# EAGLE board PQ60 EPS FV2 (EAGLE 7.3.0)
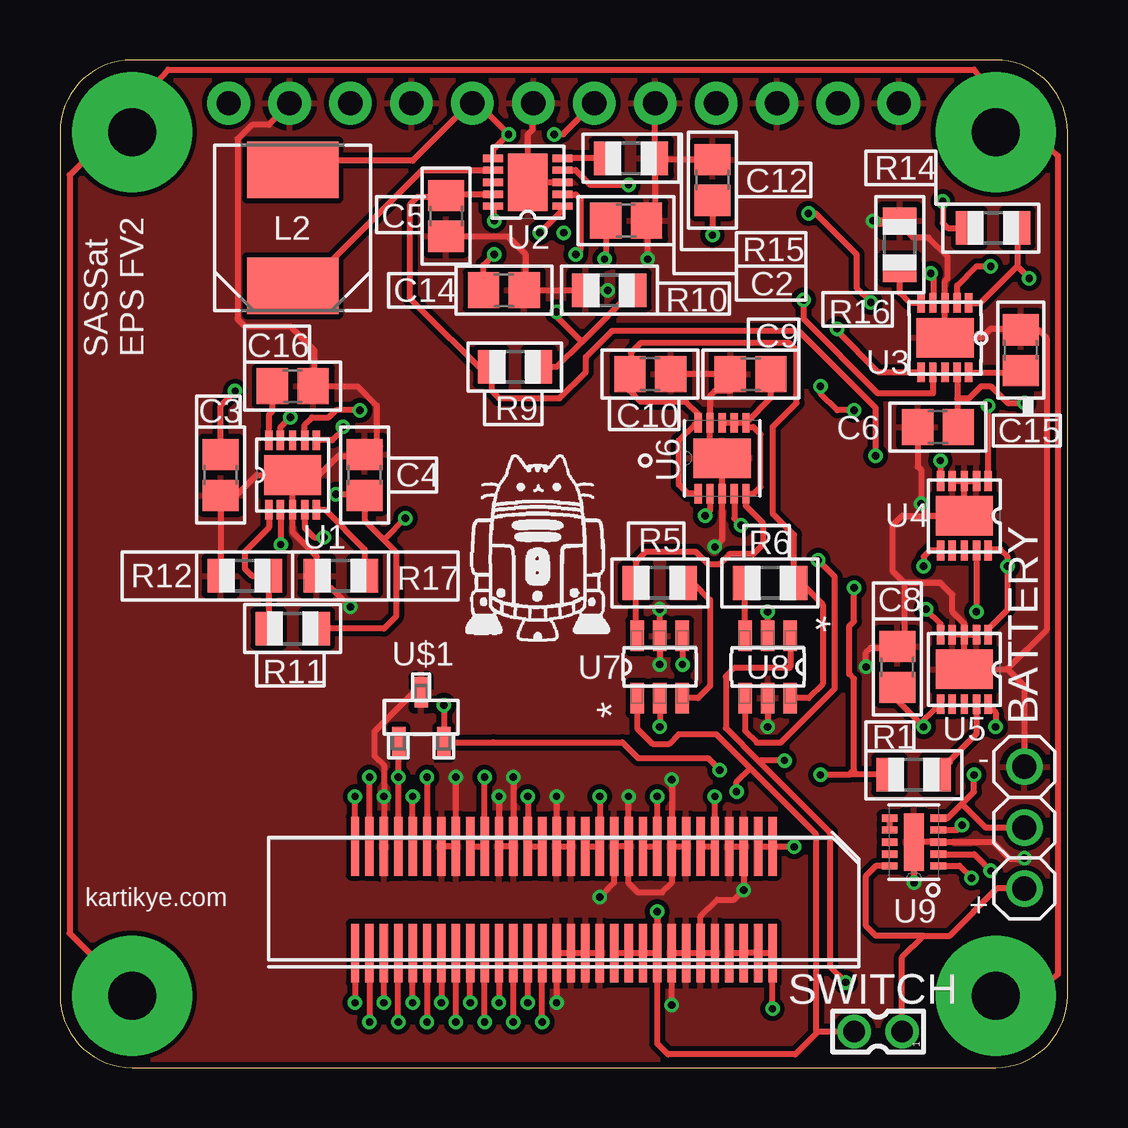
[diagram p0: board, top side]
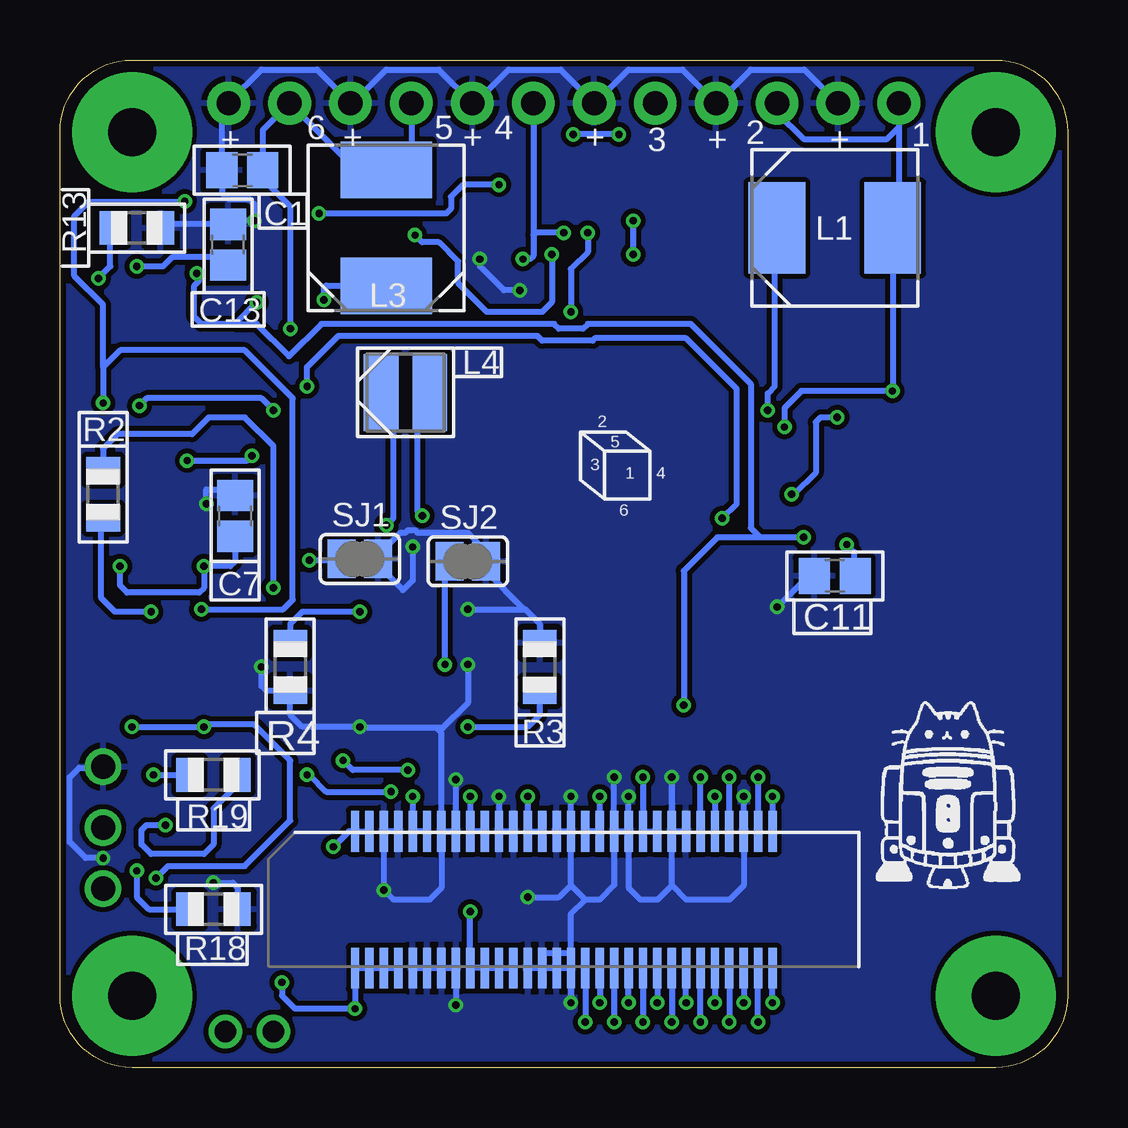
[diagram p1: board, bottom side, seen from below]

Size 42 x 42 mm. Coordinates in mm from the lower left corner, seen from the top.
Outline: 42,3 42,39 arc90 39,42 3,42 arc90 0,39 0,3 arc90 3,0 39,0 arc90 42,3
Copper layers (1*16): Top 0.035mm / dielectric 1.5mm / Bottom 0.035mm
Design rules "SeeedStudio_2layer_DRU_no_angle_20140221 *": minimum track width 6mil, minimum drill 0.3mm, track to track 6mil, track to pad 6mil, pad to pad 6mil, via to via 6mil, smd to smd 0mil, copper to edge 10mil, drill to drill 10mil, minimum pad ring 10mil, minimum via ring 6mil, stop-mask expansion 2mil, vias tented up to drill 100mil, thermal gap 10mil
Net classes: 0 default: clearance 0.205 mm

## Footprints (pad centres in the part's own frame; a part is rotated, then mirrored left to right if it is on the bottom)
1X03 = drill 1.016: 1 -2.54,0; 2 0,0; 3 2.54,0
C0805 = smd 1.3 x 1.5: 1 -0.85,0; 2 0.85,0
IND_ELL6XH = smd 2.362 x 3.81: 1 -2.413,0; 2 2.413,0
IND_ELL3FU = smd 1.448 x 3.2: 1 -1.016,0; 2 1.016,0
R0805 = smd 1.1 x 1.4: 1 -1,0; 2 1,0
SJ = smd 1.168 x 1.6: 1 -0.762,0; 2 0.762,0
1X12-CB = drill 1.016 pad 1.778: 1 -13.97,0; 2 -11.43,0; 3 -8.89,0; 4 -6.35,0; 5 -3.81,0; 6 -1.27,0; 7 1.27,0; 8 3.81,0; 9 6.35,0; 10 8.89,0; 11 11.43,0; 12 13.97,0
332-02 = drill 0.9 pad 1.27: 1 0,-1; 2 0,1
DFN300X300X80-11N = smd 0.813 x 0.305: 1 -1.448,0.991; 2 -1.448,0.508; 3 -1.448,0; 4 -1.448,-0.508; 5 -1.448,-0.991; 6 1.448,-0.991; 7 1.448,-0.508; 8 1.448,0; 9 1.448,0.508; 10 1.448,0.991 | smd 1.651 x 2.388: 11 0,0
SON50P300X300X100-11N = smd 0.813 x 0.305: 1 -1.473,0.991; 2 -1.473,0.508; 3 -1.473,0; 4 -1.473,-0.508; 5 -1.473,-0.991; 6 1.473,-0.991; 7 1.473,-0.508; 8 1.473,0; 9 1.473,0.508; 10 1.473,0.991 | smd 1.651 x 2.388: 11 0,0
SOT95P280X145-6N = smd 1.27 x 0.559: 1 -1.295,0.94; 2 -1.295,0; 3 -1.295,-0.94; 4 1.295,-0.94; 5 1.295,0; 6 1.295,0.94
SON50P200X300X80-11N = smd 0.66 x 0.305: 1 -1.016,0.991; 2 -1.016,0.508; 3 -1.016,0; 4 -1.016,-0.508; 5 -1.016,-0.991; 6 1.016,-0.991; 7 1.016,-0.508; 8 1.016,0; 9 1.016,0.508; 10 1.016,0.991 | smd 0.838 x 2.388: 11 0,0
SOT95P237X112-3N = smd 0.559 x 1.27: 1 -0.94,-1.041; 2 0.94,-1.041; 3 0,1.041
FX8C-060S-SV(92) = smd 0.35 x 1.7: P$1 -8.7,2.85; P$2 -8.1,2.85; P$3 -7.5,2.85; P$4 -6.9,2.85; P$5 -6.3,2.85; P$6 -5.7,2.85; P$7 -5.1,2.85; P$8 -4.5,2.85; P$9 -3.9,2.85; P$10 -3.3,2.85; P$11 -2.7,2.85; P$12 -2.1,2.85; P$13 -1.5,2.85; P$14 -0.9,2.85; P$15 -0.3,2.85; P$16 0.3,2.85; P$17 0.9,2.85; P$18 1.5,2.85; P$19 2.1,2.85; P$20 2.7,2.85; P$21 3.3,2.85; P$22 3.9,2.85; P$23 4.5,2.85; P$24 5.1,2.85; P$25 5.7,2.85; P$26 6.3,2.85; P$27 6.9,2.85; P$28 7.5,2.85; P$29 8.1,2.85; P$30 8.7,2.85; P$31 8.7,-2.85; P$32 8.1,-2.85; P$33 7.5,-2.85; P$34 6.9,-2.85; P$35 6.3,-2.85; P$36 5.7,-2.85; P$37 5.1,-2.85; P$38 4.5,-2.85; P$39 3.9,-2.85; P$40 3.3,-2.85; P$41 2.7,-2.85; P$42 2.1,-2.85; P$43 1.5,-2.85; P$44 0.9,-2.85; P$45 0.3,-2.85; P$46 -0.3,-2.85; P$47 -0.9,-2.85; P$48 -1.5,-2.85; P$49 -2.1,-2.85; P$50 -2.7,-2.85; P$51 -3.3,-2.85; P$52 -3.9,-2.85; P$53 -4.5,-2.85; P$54 -5.1,-2.85; P$55 -5.7,-2.85; P$56 -6.3,-2.85; P$57 -6.9,-2.85; P$58 -7.5,-2.85; P$59 -8.1,-2.85; P$60 -8.7,-2.85
FX8C-060P-SV(92) = smd 0.35 x 2.45: P$1 -8.7,-2.225; P$2 -8.1,-2.225; P$3 -7.5,-2.225; P$4 -6.9,-2.225; P$5 -6.3,-2.225; P$6 -5.7,-2.225; P$7 -5.1,-2.225; P$8 -4.5,-2.225; P$9 -3.9,-2.225; P$10 -3.3,-2.225; P$11 -2.7,-2.225; P$12 -2.1,-2.225; P$13 -1.5,-2.225; P$14 -0.9,-2.225; P$15 -0.3,-2.225; P$16 0.3,-2.225; P$17 0.9,-2.225; P$18 1.5,-2.225; P$19 2.1,-2.225; P$20 2.7,-2.225; P$21 3.3,-2.225; P$22 3.9,-2.225; P$23 4.5,-2.225; P$24 5.1,-2.225; P$25 5.7,-2.225; P$26 6.3,-2.225; P$27 6.9,-2.225; P$28 7.5,-2.225; P$29 8.1,-2.225; P$30 8.7,-2.225; P$31 8.7,2.225; P$32 8.1,2.225; P$33 7.5,2.225; P$34 6.9,2.225; P$35 6.3,2.225; P$36 5.7,2.225; P$37 5.1,2.225; P$38 4.5,2.225; P$39 3.9,2.225; P$40 3.3,2.225; P$41 2.7,2.225; P$42 2.1,2.225; P$43 1.5,2.225; P$44 0.9,2.225; P$45 0.3,2.225; P$46 -0.3,2.225; P$47 -0.9,2.225; P$48 -1.5,2.225; P$49 -2.1,2.225; P$50 -2.7,2.225; P$51 -3.3,2.225; P$52 -3.9,2.225; P$53 -4.5,2.225; P$54 -5.1,2.225; P$55 -5.7,2.225; P$56 -6.3,2.225; P$57 -6.9,2.225; P$58 -7.5,2.225; P$59 -8.1,2.225; P$60 -8.7,2.225

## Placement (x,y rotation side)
BATTERY  [1X03]  40.2,10 90 top
C1  10uF  [C0805]  34.4,37.4 0 bottom
C2  10uF  [C0805]  23.6,35.3 180 top
C3  10uF  [C0805]  6.7,24.7 90 top
C4  10uF  [C0805]  12.7,24.7 90 top
C5  10uF  [C0805]  16.1,35.5 270 top
C6  10uF  [C0805]  36.6,26.7 180 top
C7  4.7uF  [C0805]  34.7,23 270 bottom
C8  4.7uF  [C0805]  34.9,16.7 270 top
C9  10uF  [C0805]  28.79,28.9 0 top
C10  10uF  [C0805]  24.61,28.91 180 top
C11  4.7uF  [C0805]  9.7,20.5 180 bottom
C12  4.7uF  [C0805]  27.2,37 90 top
C13  4.7uF  [C0805]  35,34.3 90 bottom
C14  1uF  [C0805]  18.5,32.4 0 top
C15  1uF  [C0805]  40.05,29.9 90 top
C16  1uF  [C0805]  9.7,28.4 0 top
L1  10UH  [IND_ELL6XH]  9.7,35 0 bottom
L2  10UH  [IND_ELL6XH]  9.7,35 90 top
L3  10UH  [IND_ELL6XH]  28.4,35 90 bottom
L4  2.2UH  [IND_ELL3FU]  27.6,28.13 0 bottom
R1  470k  [R0805]  35.58,12.21 180 top
R2  470k  [R0805]  40.2,23.9 90 bottom
R3  35.7k  [R0805]  22,16.7 90 bottom
R4  35.7k  [R0805]  32.4,16.7 270 bottom
R5  35.7k  [R0805]  25,20.2 0 top
R6  35.7k  [R0805]  29.6,20.2 180 top
R9  15k  [R0805]  18.97,29.21 180 top
R10  4.7k  [R0805]  22.9,32.4 0 top
R11  15k  [R0805]  9.7,18.3 0 top
R12  4.7k  [R0805]  7.7,20.5 0 top
R13  4.7k  [R0805]  38.8,35 180 bottom
R14  15k  [R0805]  38.9,35 180 top
R15  466k  [R0805]  23.8,37.9 180 top
R16  466k  [R0805]  35,34.3 270 top
R17  466k  [R0805]  11.7,20.5 0 top
R18  487  [R0805]  35.6,6.6 180 bottom
R19  [R0805]  35.6,12.2 180 bottom
SJ1  [SJ]  29.5,21.2 180 bottom
SJ2  [SJ]  25,21.1 180 bottom
SOLAR_PANELS  [1X12-CB]  21,40.2 0 top
SWITCH  332-02  [332-02]  34.1,1.5 90 top
U1  LTC3105EDDPBF  [DFN300X300X80-11N]  9.7,24.7 90 top
U2  LTC3105EDDPBF  [DFN300X300X80-11N]  19.5,36.9 180 top
U3  LTC3105EDDPBF  [DFN300X300X80-11N]  36.89,30.42 270 top
U4  LTC4413EDDPBF  [DFN300X300X80-11N]  37.7,23 270 top
U5  LTC4413EDDPBF  [DFN300X300X80-11N]  37.7,16.6 270 top
U6  TPS63001DRCR  [SON50P300X300X100-11N]  27.6,25.4 90 top
U7  TPS2552DBVT  [SOT95P280X145-6N]  25,16.7 90 top
U8  TPS2552DBVT  [SOT95P280X145-6N]  29.5,16.7 270 top
U9  BQ24210DQCT  [SON50P200X300X80-11N]  35.6,9.4 180 top
U$1  MCP130T-315I/TT  [SOT95P237X112-3N]  15.06,14.6 0 top
U$2  FX8C-060S-SV(92)  [FX8C-060S-SV(92)]  21,7 0 bottom
U$3  FX8C-060P-SV(92)  [FX8C-060P-SV(92)]  21,7 180 top

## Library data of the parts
BATTERY C1-C16 R1-R6 R9-R19 SOLAR_PANELS = adafruit
L1-L3 = Panasonic-ELL; MPN: ELL6SH100M; OC_FARNELL: 1539555; OC_NEWARK: 95M4201; PACKAGE: SMD; SUPPLIER: PANASONIC
L4 = Panasonic-ELL; CURRENTRATING: 1.6A; MPN: ELL3FU2R2N; OC_FARNELL: 1888686; OC_NEWARK: 56T0899; PACKAGE: SMD-3FU; SUPPLIER: PANASONIC; TOLERANCE: ±30 %
SJ1 SJ2 = jumper
SWITCH = con-garry
U1-U3 = LTC3105; MPN: LTC3105EDD#PBF; OC_FARNELL: 1898600; OC_NEWARK: 27T5809; PACKAGE: DFN-10; SUPPLIER: Linear Technology
U4 U5 = LTC4413; MPN: LTC4413EDD#PBF; OC_FARNELL: 1663736; OC_NEWARK: 56M9529; PACKAGE: DFN-10; SUPPLIER: Linear Technology
U6 = TPS63001; MPN: TPS63001DRCR; OC_FARNELL: -; OC_NEWARK: 85K1711; PACKAGE: SON-10; SUPPLIER: TEXAS INSTRUMENTS
U7 U8 = TPS2552; MPN: TPS2552DBVT; OC_FARNELL: 1694421; OC_NEWARK: 40P3866; PACKAGE: SOT-23-6; SUPPLIER: Texas Instruments
U9 = BQ24210; MPN: BQ24210DQCT; OC_FARNELL: 1903633; OC_NEWARK: 56T0491; PACKAGE: SON-10; SUPPLIER: TEXAS INSTRUMENTS
U$1 = MCP130T; MPN: MCP130T-315I/TT; OC_FARNELL: 3021154; OC_NEWARK: 96K3703; PACKAGE: SOT-3; SUPPLIER: Microchip
U$2 U$3 = PQ60

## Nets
!RST: U$1.1 U$2.P$27 U$3.P$27
+3V3: U1.4 U2.4 U3.4 U8.1 U$1.2 U$2.P$57 U$2.P$58 U$2.P$59 U$2.P$60 U$3.P$57 U$3.P$58 U$3.P$59 U$3.P$60
+3V3_SW1: U$2.P$1 U$2.P$2 U$3.P$1 U$3.P$2
+3V3_SW2: U$2.P$5 U$2.P$6 U$3.P$5 U$3.P$6
+3V3_SW3: U$2.P$9 U$2.P$10 U$3.P$9 U$3.P$10
BATTERY: C9.2 R5.1 U6.5 U6.6 U6.7 U6.8 U7.6
BATV: R1.2 R2.2 SWITCH.2 U7.1 U$2.P$49 U$2.P$50 U$2.P$51 U$2.P$52 U$3.P$49 U$3.P$50 U$3.P$51 U$3.P$52
BATV_SW1: U$2.P$13 U$2.P$14 U$3.P$13 U$3.P$14
BATV_SW2: U$2.P$17 U$2.P$18 U$3.P$17 U$3.P$18
BATV_SW3: U$2.P$21 U$2.P$22 U$3.P$21 U$3.P$22
GND: BATTERY.3 C1.1 C2.1 C3.1 C4.2 C5.2 C6.2 C7.1 C8.1 C9.1 C10.1 C11.2 C12.2 C13.2 C14.2 C15.2 C16.2 R3.2 R4.2 R10.1 R12.1 R13.1 R15.1 R16.1 R17.1 R18.1 SJ1.1 SJ2.1 SOLAR_PANELS.2 SOLAR_PANELS.4 SOLAR_PANELS.6 SOLAR_PANELS.8 SOLAR_PANELS.10 SOLAR_PANELS.12 U1.3 U1.11 U2.3 U2.11 U3.3 U3.11 U4.2 U4.3 U4.4 U4.11 U5.2 U5.3 U5.4 U5.11 U6.3 U6.9 U6.11 U7.5 U8.5 U9.3 U9.11 U$1.3 U$2.P$3 U$2.P$4 U$2.P$7 U$2.P$8 U$2.P$11 U$2.P$12 U$2.P$15 U$2.P$16 U$2.P$19 U$2.P$20 U$2.P$23 U$2.P$24 U$2.P$28 U$2.P$45 U$2.P$46 U$2.P$47 U$2.P$48 U$2.P$53 U$2.P$54 U$2.P$55 U$2.P$56 U$3.P$3 U$3.P$4 U$3.P$7 U$3.P$8 U$3.P$11 U$3.P$12 U$3.P$15 U$3.P$16 U$3.P$19 U$3.P$20 U$3.P$23 U$3.P$24 U$3.P$28 U$3.P$45 U$3.P$46 U$3.P$47 U$3.P$48 U$3.P$53 U$3.P$54 U$3.P$55 U$3.P$56
GPIO0: U$2.P$25 U$3.P$25
GPIO1: U$2.P$26 U$3.P$26
GPIO2: U$2.P$34 U$3.P$34
GPIO3: U$2.P$35 U$3.P$35
GPIO4: U$2.P$36 U$3.P$36
GPIO5: U$2.P$37 U$3.P$37
GPIO6: U$2.P$38 U$3.P$38
GPIO7: U$2.P$39 U$3.P$39
GPIO8: U$2.P$40 U$3.P$40
GPIO9: U$2.P$41 U$3.P$41
GPIO10: U$2.P$42 U$3.P$42
GPIO11: U$2.P$43 U$3.P$43
GPIO12: U$2.P$44 U$3.P$44
MISO: U$2.P$32 U$3.P$32
MOSI: U$2.P$31 U$3.P$31
N$1: L2.1 U2.7
N$2: L3.1 U3.7
N$3: L1.1 U1.7
N$4: L4.1 U6.4
N$5: C4.1 R11.2 U1.9 U4.1
N$6: C5.1 R9.2 U2.9 U4.5
N$7: C6.1 R14.2 U3.9 U5.5
N$8: R4.1 U8.2
N$9: C7.2 U4.6 U4.10 U5.1
N$10: R1.1 U5.9
N$11: R2.1 U4.9
N$12: L4.2 U6.2
N$13: R3.1 U7.2
N$14: R5.2 U7.3
N$15: R6.2 U8.3
N$16: SJ1.2 U8.4
N$17: SJ2.2 U7.4
N$18: R13.2 R14.1 U3.1
N$19: C11.1 U1.2
N$20: C12.1 U2.2
N$21: C13.1 U3.2
N$22: C14.1 U2.10
N$23: C15.1 U3.10
N$24: C16.1 U1.10
N$25: R11.1 R12.2 U1.1
N$26: R9.1 R10.2 U2.1
N$28: R15.2 U2.5
N$29: R16.2 U3.5
N$30: R17.2 U1.5
N$31: C8.2 U5.6 U5.10 U9.1
N$32: U9.6 U9.7
N$33: R18.2 U9.2
N$34: BATTERY.1 SWITCH.1 U9.10
N$35: BATTERY.2 R19.2 U9.5
N$36: R19.1 U9.4
PANEL1+2: C3.2 L1.2 SOLAR_PANELS.1 SOLAR_PANELS.3 U1.6
PANEL3+4: C2.2 L2.2 SOLAR_PANELS.5 SOLAR_PANELS.7 U2.6
PANEL5+6: C1.2 L3.2 SOLAR_PANELS.9 SOLAR_PANELS.11 U3.6
SCK: U$2.P$33 U$3.P$33
SCL: U$2.P$29 U$3.P$29
SDA: U$2.P$30 U$3.P$30
UNPROTECTED3V3: C10.2 R6.1 U6.1 U6.10 U8.6

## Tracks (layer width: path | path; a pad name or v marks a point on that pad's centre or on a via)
!RST  (via drill 0.3)
  Top 0.254: U$3.P$27 v14.1,12.1 U$1.1
  Bottom 0.254: U$2.P$27 v14.1,12.1
+3V3  (via drill 0.3)
  Top 0.254: U$3.P$57 U$3.P$58 U$3.P$59 U$3.P$60 v29.7,2.45 | U8.1 30.44,16.69 30.4,16.65 28.1,16.65 27.75,16.3 27.75,14.15 29.15,12.75 | 29.15,12.75 32.1,9.8 32.1,4.2 v32.75,3.55 | U$1.2 18.06,13.56 | v30.2,12.8 29.2,12.8 29.15,12.75 | 27.3,12.6 v27.5,12.4 27,12.9 24.1,12.9 23.44,13.56 U$1.2 | v16,15.1 U$1.2 | U$1.2 | U2.4 21.49,37.41 22.1,36.8 v23.7,36.8 | v31.2,35.6 31.5,35.6 33.2,33.9 33.2,32.5 v33.8,31.9 | U3.4 36.4,31.89 36.4,32.9 v36.3,33.1 | U1.4 10.21,22.51 10.2,22.5 10.6,22.1 v11,22.1
  Bottom 0.254: U$2.P$60 U$2.P$59 U$2.P$58 U$2.P$57 | v32.75,3.55 32.75,3 32.2,2.45 v29.7,2.45 U$2.P$60 | U$2.P$60 U$3.P$60 | v27.5,12.4 29.8,12.4 v30.2,12.8 | v11,22.1 12.8,22.1 | 12.8,22.1 14.6,22.1 16,20.7 v16,15.1 | v23.7,36.8 25.2,36.8 25.7,36.3 25.7,35.8 25.9,35.6 v31.2,35.6 | v33.8,31.9 34.7,31 | 34.7,31 36.1,31 36.4,31.3 36.4,32.6 36.2,32.8 v36.3,33.1 | 34.7,31 33.8,31 32.45,29.65 31.1,31 21.4,31 21.2,30.8 20.2,30.8 20,31 15.7,31 13.2,28.5 13.2,22.5 12.8,22.1
+3V3_SW1  (via drill 0.3)
  Top 0.254: v30.6,9.2 29.73,9.2 U$3.P$1 U$3.P$2
  Bottom 0.254: U$2.P$2 U$2.P$1 29.95,9.85 v30.6,9.2
+3V3_SW2  (via drill 0.3)
  Top 0.254: U$3.P$6 U$3.P$5 v27.3,11.3
  Bottom 0.254: U$2.P$6 U$2.P$5 v27.3,11.3
+3V3_SW3  (via drill 0.3)
  Top 0.254: U$3.P$10 U$3.P$9 v24.9,11.3
  Bottom 0.254: U$2.P$10 U$2.P$9 | v24.9,11.3 U$2.P$9 | 24.9,9.1 U$2.P$9
BATTERY
  Top 0.254: 24.1,18 U7.6 24,18 R5.1 24,21.1 24.4,21.5 26.5,21.5 27,21 27.5,21 27.9,21.4 28.9,21.4 29.3,21.8 29.3,22.7 28.59,23.41 U6.5 28.93,23.93 29.2,24.2 29.2,26.4 28.9,26.7 28.7,26.7 28.59,26.81 U6.6 | U6.6 U6.7 U6.8 | U6.6 29.64,27.92 C9.2
BATV  (via drill 0.3)
  Top 0.254: U$3.P$49 U$3.P$50 U$3.P$51 U$3.P$52 | U7.1 24.06,14.14 24.7,13.5 25.4,13.5 25.8,13.9 27.35,13.9 28.77,12.47 | 28.77,12.47 31.5,9.75 31.5,1.4 | 31.5,1.4 30.65,0.55 25.35,0.55 24.9,1 v24.9,6.5 U$3.P$52 | 24.85,4.72 U$3.P$52 | R1.2 32.91,12.21 | v31.7,12.2 v31.71,12.21 32.91,12.21 | v28.2,11.5 28.2,11.9 28.77,12.47 | SWITCH.2 31.6,1.5 31.5,1.4 | 32.91,12.21 33.1,12.4 33.1,16.2 32.9,16.4 32.9,18.4 33.1,18.6 v33.1,20
  Bottom 0.254: U$2.P$49 U$2.P$50 U$2.P$51 U$2.P$52 v24.9,6.5 | v31.7,12.2 31.6,12.2 30.9,11.5 v28.2,11.5 | R2.2 40.2,25.8 39.6,26.4 36.5,26.4 35.8,27.1 34.3,27.1 33.1,25.9 v33.1,20
BATV_SW1  (via drill 0.3)
  Top 0.254: U$3.P$14 U$3.P$13 v22.5,11.3
  Bottom 0.254: U$2.P$14 U$2.P$13 v22.5,11.3
BATV_SW2  (via drill 0.3)
  Top 0.254: U$3.P$17 U$3.P$18 v19.5,11.3
  Bottom 0.254: U$2.P$17 U$2.P$18 v19.5,11.3
BATV_SW3  (via drill 0.3)
  Top 0.254: U$3.P$22 U$3.P$21 v17.7,12.1
  Bottom 0.254: U$2.P$22 U$2.P$21 v17.7,12.1
CHASSIS_GND  (via drill 2 pad 5)
  Top 0.254: v3,3 0.4,5.6 0.4,37.2 2.2,39 v3,39 3,40 4.5,41.6 38.1,41.6 39,40.6 v39,39 40.5,39 41.6,38 41.6,3.9 40.6,3 v39,3
GND  (via drill 0.3, 0.3 pad 0.45)
  Top 0.254: U$3.P$48 U$3.P$47 U$3.P$46 U$3.P$45 v20.7,2.7 | U$3.P$55 U$3.P$54 U$3.P$53 v25.5,2.6 | U$3.P$55 U$3.P$56 | v25,19.1 U7.5 v25,16.8 | U8.5 v29.5,14.2 | U6.9 27.1,25.7 27.4,25.4 U6.11 U6.3 27.6,22 v27.3,21.7 | U6.9 27.09,27.34 | C10.1 C9.1 27.95,28.2 27.3,28.2 27.1,28 27.1,26.88 U6.9 | U5.3 U5.11 39.48,16.62 | U5.3 U5.4 | U5.3 U5.2 | 39.48,16.62 40.2,15.9 BATTERY.3 | v35.6,7.7 U9.11 U9.3 38.9,9.4 39.6,8.7 40.17,8.7 v40.2,8.73 | v33.6,16.7 33.6,17.3 33.8,17.5 34.75,17.5 C8.1 35.2,17.85 35.2,20.2 | U4.3 U4.11 36.1,23 | U4.3 U4.2 | U4.3 U4.4 | 35.2,20.2 34.7,20.7 34.7,22.6 35.1,23 36.1,23 | 36.1,23 36.1,23.3 v35.9,23.5 35.9,24.9 35.75,25.05 C6.2 | U5.3 37.7,18.5 37.2,19 37.2,19.7 36.7,20.2 35.2,20.2 | R16.1 v33.9,35.3 34.05,35.15 C13.2 35.55,34.6 36.2,34.6 37,33.8 37,32.9 36.89,32.79 U3.3 U3.11 38.42,30.42 38.8,30.8 40,30.8 C15.2 40.78,30.75 41.13,30.4 41.13,18.24 39.48,16.62 | U1.11 U1.3 9.7,22.3 10.7,21.3 R17.1 11.2,20 11.3,20 v12.1,19.2 | U1.11 10.8,24.7 11.6,25.5 12.65,25.5 C4.2 13.2,26.05 | U1.11 8.2,24.7 7.35,23.85 C3.1 R12.1 | 13.2,26.05 13.2,27.6 12.4,28.4 C16.2 10.6,28.45 10.6,29.9 9.6,30.9 7.7,30.9 7.4,31.2 7.4,38.7 8,39.3 8.7,39.3 9.57,40.17 SOLAR_PANELS.2 | C5.2 18.65,34.65 19.4,33.9 19.4,32.45 C14.2 R10.1 | 22.7,32.4 R10.1 | U2.3 U2.11 19.5,38.9 19.7,39.1 19.7,40.17 SOLAR_PANELS.6 | R10.1 v22.83,32.4 | v24.5,33.7 24.5,35.25 C2.1 24.8,35.65 R15.1 | C12.2 24.85,37.85 R15.1 | R15.1 SOLAR_PANELS.8 | 13.35,25.9 13.2,26.05 | U$3.P$28 v13.5,11.3 13.5,12.6 13.1,13 13.1,14 14.74,15.64 U$1.3 | U$3.P$24 U$3.P$23 v16.5,12.1 | v18.3,11.3 U$3.P$20 U$3.P$19 v18.9,12.1 | U$3.P$15 U$3.P$16 v20.7,11.3
  Top 0.254: U$3.P$11 U$3.P$12 23.1,7.7 v22.5,7.1 | U$3.P$8 U$3.P$7 | U$3.P$11 v23.7,11.3 | U$3.P$4 U$3.P$3 v28.5,7.4 28.1,7 27.4,7 26.7,6.3 U$3.P$55 | v25.5,12 U$3.P$8 | U$3.P$8 25.5,7.7 25.1,7.3 24.1,7.3 23.7,7.7 U$3.P$11
  Bottom 0.254: U$2.P$24 U$2.P$23 v16.5,12.1 16.5,7.6 | U$2.P$19 U$2.P$20 | U$2.P$15 U$2.P$16 | U$2.P$12 U$2.P$11 v23.7,11.3 | U$2.P$7 U$2.P$8 v25.5,12 | U$2.P$4 U$2.P$3 v28.5,7.4 28.1,7 26.6,7 26.1,7.5 U$2.P$7 | U$2.P$48 U$2.P$47 U$2.P$46 U$2.P$45 v20.7,2.7 U$3.P$45 | U$2.P$56 U$2.P$55 U$2.P$54 U$2.P$53 v25.5,2.6 | v25,19.1 22.65,19.1 | 22.65,19.1 22.6,19.1 22,18.5 R3.2 | 22.65,19.1 24.24,20.69 SJ2.1 24.45,21.31 24.45,21.75 25,22.3 27.1,22.3 27.2,22.4 27.5,22.4 27.6,22.3 27.8,22.3 28.64,21.46 28.74,21.46 SJ1.1 28.74,20.94 27.7,19.9 27.3,20.3 v27.3,21.7 | v25,16.8 25,15.2 26.05,14.15 26.3,14.15 | 26.3,14.15 29.45,14.15 v29.5,14.2 31.9,14.2 32.4,14.7 R4.2 33.4,15.7 33.6,15.9 v33.6,16.7 | U$2.P$7 26.1,13.95 26.3,14.15 | v35.6,7.7 34.8,7.7 34.6,7.5 R18.1 | v35.9,23.5 35.9,24.1 34.95,24.1 C7.1 | SOLAR_PANELS.2 10.97,41.6 13.2,41.6 14.6,40.2 SOLAR_PANELS.4 16.05,41.6 18.3,41.6 19.7,40.2 SOLAR_PANELS.6 21.13,41.6 23.3,41.6 24.7,40.2 SOLAR_PANELS.8 26.21,41.6 28.4,41.6 29.8,40.2 SOLAR_PANELS.10 31.29,41.6 33.6,41.6 34.97,40.23 SOLAR_PANELS.12 35.25,39.92 C1.1 35.25,36.45 35,36.2 34.1,36.2 33.9,36 v33.9,35.3 34.85,35.3 C13.2 37.65,35.15 R13.1 | v22.83,32.4 23.5,32.4 24.5,33.4 v24.5,33.7 | BATTERY.3 40.24,12.5 41.2,12.5 41.6,12.1 41.6,9.4 40.93,8.73 v40.2,8.73 | v13.5,11.3 U$2.P$28 13.5,7.6 14.1,7 15.9,7 16.5,7.6 | U$2.P$20 v18.3,11.3 | U$2.P$19 v18.9,12.1 | U$2.P$20 18.3,7.5 17.8,7 17.1,7 16.5,7.6 | U$2.P$19 18.9,7.6 19.5,7 20.1,7 | 20.7,7.6 U$2.P$16 | U$2.P$16 v20.7,11.3 | 20.1,7 20.7,7.6 | U$3.P$47 U$3.P$45 | U$3.P$45 20.7,6.4 20.1,7 | v22.5,7.1 21.2,7.1 20.7,7.6 | C11.2 10.8,20.5 v12.1,19.2
  pour Top: 39.1,42 3.1,42 arc90 0,38.9 0,3.3 arc90 3.3,0 38.8,0 arc90 42,3.2 42,39.1 arc90
  pour Bottom: 25.8,42 3.1,42 arc90 0,38.9 0,3.1 arc90 3.2,-0.1 38.8,-0.1 arc90 42,3.1 42,39.1 arc90 39.1,42 26.1,42
GPIO0  (via drill 0.3)
  Top 0.254: v15.3,12.1 U$3.P$25
  Bottom 0.254: U$2.P$25 v15.3,12.1
GPIO1  (via drill 0.3)
  Top 0.254: U$3.P$26 v14.7,11.3
  Bottom 0.254: v14.7,11.3 U$2.P$26
GPIO2  (via drill 0.3)
  Top 0.254: v14.1,1.9 U$3.P$34
  Bottom 0.254: U$2.P$34 v14.1,1.9
GPIO3  (via drill 0.3)
  Top 0.254: v14.7,2.7 U$3.P$35
  Bottom 0.254: U$2.P$35 v14.7,2.7
GPIO4  (via drill 0.3)
  Top 0.254: U$3.P$36 v15.3,1.9
  Bottom 0.254: v15.3,1.9 U$2.P$36
GPIO5  (via drill 0.3)
  Top 0.254: U$3.P$37 v15.9,2.7
  Bottom 0.254: v15.9,2.7 U$2.P$37
GPIO6  (via drill 0.3)
  Top 0.254: v16.5,1.9 U$3.P$38
  Bottom 0.254: U$2.P$38 v16.5,1.9
GPIO7  (via drill 0.3)
  Top 0.254: v17.1,2.7 U$3.P$39
  Bottom 0.254: U$2.P$39 v17.1,2.7
GPIO8  (via drill 0.3)
  Top 0.254: v17.7,1.9 U$3.P$40
  Bottom 0.254: U$2.P$40 v17.7,1.9
GPIO9  (via drill 0.3)
  Top 0.254: U$3.P$41 v18.3,2.7
  Bottom 0.254: v18.3,2.7 U$2.P$41
GPIO10  (via drill 0.3)
  Top 0.254: v18.9,1.9 U$3.P$42
  Bottom 0.254: U$2.P$42 v18.9,1.9
GPIO11  (via drill 0.3)
  Top 0.254: v19.5,2.7 U$3.P$43
  Bottom 0.254: U$2.P$43 v19.5,2.7
GPIO12  (via drill 0.3)
  Top 0.254: v20.1,1.9 U$3.P$44
  Bottom 0.254: U$2.P$44 v20.1,1.9
MISO  (via drill 0.3)
  Top 0.254: U$3.P$32 v12.9,1.9
  Bottom 0.254: v12.9,1.9 U$2.P$32
MOSI  (via drill 0.3)
  Top 0.254: U$3.P$31 v12.3,2.7
  Bottom 0.254: v12.3,2.7 U$2.P$31
N$1
  Top 0.254: U2.7 15.1,37.4 10.29,32.59 L2.1
N$2  (via drill 0.3)
  Top 0.254: U3.7 36.38,28.12 36.4,28.1 34.1,28.1 31,31.2 v31,32
  Bottom 0.254: v31,32 31,32.5 30.9,32.6 28.47,32.6 L3.1
N$3  (via drill 0.3)
  Top 0.254: v12.5,27.4 11.5,27.4 11.2,27.1 10.5,27.1 10.2,26.8 U1.7
  Bottom 0.254: v12.5,27.4 12.5,28.1 12.2,28.4 12.2,34.91 L1.1
N$4  (via drill 0.3)
  Top 0.254: U6.4 28.11,22.89 v28.4,22.6
  Bottom 0.254: v28.4,22.6 28.1,22.9 28.1,27.61 L4.1
N$5  (via drill 0.3)
  Top 0.254: U4.1 v38.69,27.59 v38.7,27.6 | 13.5,22 12.7,22.8 C4.1 12.65,23.9 v11.5,23.9 | 13.5,22 14,21.5 14,18.8 13.5,18.3 R11.2 | U1.9 9.19,26.69 v9.6,27.1 | v33.1,27.4 32.4,27.4 31.7,28.1 v31.7,28.4 | v14.4,22.9 13.5,22
  Bottom 0.254: v38.69,27.59 38.38,27.9 33.6,27.9 v33.1,27.4 | v14.4,22.9 13.8,23.5 13.8,28.3 15.9,30.4 19.7,30.4 19.8,30.3 21.9,30.3 22.1,30.5 30.4,30.5 31.7,29.2 v31.7,28.4 | v9.6,27.1 10.3,27.1 10.5,26.9 10.5,24.8 11.4,23.9 v11.5,23.9
N$6  (via drill 0.3)
  Top 0.254: v34,25.5 34,27.5 30.8,30.7 23,30.7 21.92,29.62 21.92,28.99 20.83,27.9 18.3,27.9 18,28.2 18,28.66 | U4.5 v36.71,25.29 v36.7,25.3 | U2.9 16.14,36.39 C5.1 16.05,36.3 14.9,36.3 14.6,36 14.6,32.06 18,28.66 | 17.69,29.21 R9.2 18,29.18 18,28.66
  Bottom 0.254: v36.7,25.3 34.2,25.3 v34,25.5
N$7  (via drill 0.3)
  Top 0.254: C6.1 37.4,26.75 U3.9 37.4,27.9 37.9,27.9 38.4,28.4 38.8,28.4 39.5,27.7 v40.2,27.7 | U5.5 36.71,18.49 v36.1,19.1 | v36.8,36.1 36.8,35.2 37,35 R14.2
  Bottom 0.254: 40.2,29.2 40.2,31.8 41.4,33 41.4,35.5 40.8,36.1 v36.8,36.1 | v36.1,19.1 32.7,19.1 32.3,19.5 32.3,27.9 34.3,29.9 39.5,29.9 40.2,29.2 | 40.2,29.2 v40.2,27.7
N$8  (via drill 0.3)
  Top 0.254: U8.2 v29.5,19
  Bottom 0.254: v29.5,19 31.9,19 32.4,18.5 R4.1
N$9  (via drill 0.3)
  Top 0.254: U4.6 36.25,21.55 36,21.3 v36,20.9 | U4.10 38.74,21.6 39.2,21.6 39.5,21.3 v39.5,20.9 39.5,19.1 38.69,18.29 U5.1
  Bottom 0.254: C7.2 34.7,21.1 34.9,20.9 v36,20.9 36,20 36.2,19.8 39.2,19.8 39.5,20.1 v39.5,20.9
N$10
  Top 0.254: R1.1 37.1,12.73 37.1,12.8 38.21,13.91 U5.9
N$11  (via drill 0.3)
  Top 0.254: U4.9 v38.21,19.01 v38.2,19
  Bottom 0.254: v38.2,19 39.7,19 40.3,19.6 40.3,22.8 R2.1 40.1,22.8
N$12  (via drill 0.3)
  Top 0.254: U6.2 27.09,23.19 v26.9,23
  Bottom 0.254: v26.9,23 27.1,23.2 27.1,27.61 L4.2
N$13  (via drill 0.3)
  Top 0.254: U7.2 v25,14.2
  Bottom 0.254: v25,14.2 22.5,14.2 22,14.7 R3.1
N$14
  Top 0.254: R5.2 26.4,20.2 27.1,19.5 27.1,15.9 26.6,15.4 U7.3
N$15
  Top 0.254: U8.3 28.56,20.16 R6.2
N$16  (via drill 0.3)
  Top 0.254: U8.4 28.56,14.04 29.05,13.55 30.05,13.55 32.3,15.8 32.3,20.45 v31.6,21.15
  Bottom 0.254: v31.6,21.15 30.31,21.15 SJ1.2
N$17  (via drill 0.3)
  Top 0.254: U7.4 v25.94,16.81 v25.95,16.8
  Bottom 0.254: v25.95,16.8 25.95,20.91 SJ2.2
N$18  (via drill 0.3)
  Top 0.254: U3.1 38.37,31.87 39.9,33.4 | R14.1 39.9,33.4 | 39.9,33.4 v40.4,32.9
  Bottom 0.254: 40.2,35.4 R13.2 39.9,34.9 39.9,33.4 v40.4,32.9
N$19  (via drill 0.3)
  Top 0.254: U1.2 v9.19,21.81 v9.2,21.8
  Bottom 0.254: v9.2,21.8 8.9,21.5 8.9,20.55 C11.1
N$20  (via drill 0.3)
  Top 0.254: U2.2 21.51,36.39 21.7,36.2 21.7,34.1 v21.5,33.9 | C12.1 v27.2,34.7
  Bottom 0.254: v21.5,33.9 21.5,31.9 21.9,31.5 24.2,31.5 25.4,32.7 25.4,33.6 26.2,34.4 26.9,34.4 v27.2,34.7
N$21  (via drill 0.3)
  Top 0.254: U3.2 37.4,32.6 38.2,33.4 v38.8,33.4
  Bottom 0.254: 35.05,33.4 C13.1 35.35,33.8 37.3,33.8 37.7,33.4 v38.8,33.4
N$22  (via drill 0.3)
  Top 0.254: C14.1 17.65,33.45 v18.1,33.9 | v18.1,35.3 18.1,35.86 U2.10
  Bottom 0.254: v18.1,33.9 v18.1,35.3
N$23
  Top 0.254: U3.10 40.02,28.97 C15.1
N$24
  Top 0.254: C16.1 8.85,27.35 8.7,27.2 U1.10
N$25
  Top 0.254: U1.1 8.71,22.51 7.7,21.5 7.7,20.8 8,20.5 R12.2 R11.1
N$26  (via drill 0.3)
  Top 0.254: R9.1 20.71,29.21 21.75,30.25 | 21.75,30.25 R10.2 | U2.1 20.95,35.75 v20,34.8 | v20.7,31.5 20.7,31.3 21.75,30.25
  Bottom 0.254: v20,34.8 20,34 20.7,33.3 v20.7,31.5
N$28
  Top 0.254: R15.2 U2.5
N$29
  Top 0.254: U3.5 35.43,31.87 35,32.3 R16.2
N$30
  Top 0.254: U1.5 11.05,23.25 12.7,21.6 R17.2
N$31  (via drill 0.3)
  Top 0.254: U5.6 36,14.48 v36,14.2 34.9,15.3 C8.2 | U9.1 37.49,8.41 v38,7.9 | U5.10 38.69,15.11 39,14.8 v39,14.2
  Bottom 0.254: v39,14.2 v36,14.2 35.9,14.3 33.9,14.3 32.4,12.8 32.4,10.3 34.3,8.4 37.5,8.4 v38,7.9
N$32
  Top 0.254: U9.7 U9.6
N$33  (via drill 0.3)
  Top 0.254: U9.2 38.11,8.89 v38.8,8.2
  Bottom 0.254: v38.8,8.2 38.8,7.1 38.3,6.6 R18.2
N$34
  Top 0.254: 36,5.5 34,5.5 33.6,5.9 33.6,8 34,8.4 U9.10 | SWITCH.1 35.1,4.6 36,5.5 | 36,5.5 37.1,5.5 39.06,7.46 BATTERY.1
N$35  (via drill 0.3)
  Top 0.254: BATTERY.2 38.6,10 37.6,11 | U9.5 36.99,10.39 37.6,11 | 37.6,11 38.1,11.5 v38.1,12.2
  Bottom 0.254: v38.1,12.2 R19.2
N$36  (via drill 0.3)
  Top 0.254: U9.4 37.4,9.9 v37.6,10.1
  Bottom 0.254: R19.1 34.6,11.8 35.6,10.8 35.6,9.3 36,8.9 38.2,8.9 38.6,9.3 38.6,9.9 38.4,10.1 v37.6,10.1
PANEL1+2  (via drill 0.3)
  Top 0.254: C3.2 6.7,27.6 v7.3,28.2 | v11.8,26.7 11.8,26.6 11.35,26.15 U1.6
  Bottom 0.254: SOLAR_PANELS.1 7.03,39.2 | SOLAR_PANELS.3 12.11,39.81 11,38.7 7.53,38.7 7.03,39.2 | v11.8,26.7 11.8,27.5 11.1,28.2 v7.3,28.2 7.29,28.21 L1.2 7.03,35.26 7.03,39.2
PANEL3+4  (via drill 0.3)
  Top 0.254: v20.6,38.9 20.97,38.9 SOLAR_PANELS.7 | L2.2 10.09,37.8 14.7,37.8 17.1,40.2 SOLAR_PANELS.5 17.4,40.2 v18.7,38.9 18.05,38.25 U2.6 | C2.2 22.75,33.75 | 22.75,33.75 v22.7,33.7 | 22.75,33.75 22.75,33.55 | 20.95,34.85 v21,34.8
  Bottom 0.254: v18.7,38.9 v20.6,38.9 | SOLAR_PANELS.7 22.27,34.7 | 22.27,34.7 22.27,33.83 22.4,33.7 v22.7,33.7 | v21,34.8 22.17,34.8 22.27,34.7
PANEL5+6  (via drill 0.3)
  Top 0.254: v32.4,30.8 32.4,30.7 34.1,29 35.87,29 U3.6
  Bottom 0.254: SOLAR_PANELS.9 27.35,38.54 L3.2 29.6,37.37 SOLAR_PANELS.11 33.55,39.08 C1.2 33.55,37.05 32.4,35.9 v32.4,30.8
SCK  (via drill 0.3)
  Top 0.254: v13.5,2.7 U$3.P$33
  Bottom 0.254: U$2.P$33 v13.5,2.7
SCL  (via drill 0.3)
  Top 0.254: U$3.P$29 v12.9,12.1
  Bottom 0.254: v12.9,12.1 U$2.P$29
SDA  (via drill 0.3)
  Top 0.254: U$3.P$30 v12.3,11.3
  Bottom 0.254: v12.3,11.3 U$2.P$30
UNPROTECTED3V3
  Top 0.254: U8.6 31.2,15.4 31.8,16 31.8,19.3 30.9,20.2 R6.1 30.6,22.2 29.7,23.1 29.7,26.7 30.7,27.7 30.7,29.9 30.4,30.2 24.2,30.2 23.8,29.8 23.8,28.95 C10.2 23.75,28.2 24.2,27.75 26.1,27.75 26.61,27.24 U6.10 26.61,26.81 26.46,26.81 25.8,26.15 25.8,24.3 26.17,23.93 U6.1 26.61,23.99

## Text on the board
tPlace: SASSat / EPS FV2 | kartikye.com
bPlace: 4 | 5 | 6 | 1 | + | 2 | + | 3 | + | + | + | + | 2 | 5 | 4 | 1 | 3 | 6
tNames: - | +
